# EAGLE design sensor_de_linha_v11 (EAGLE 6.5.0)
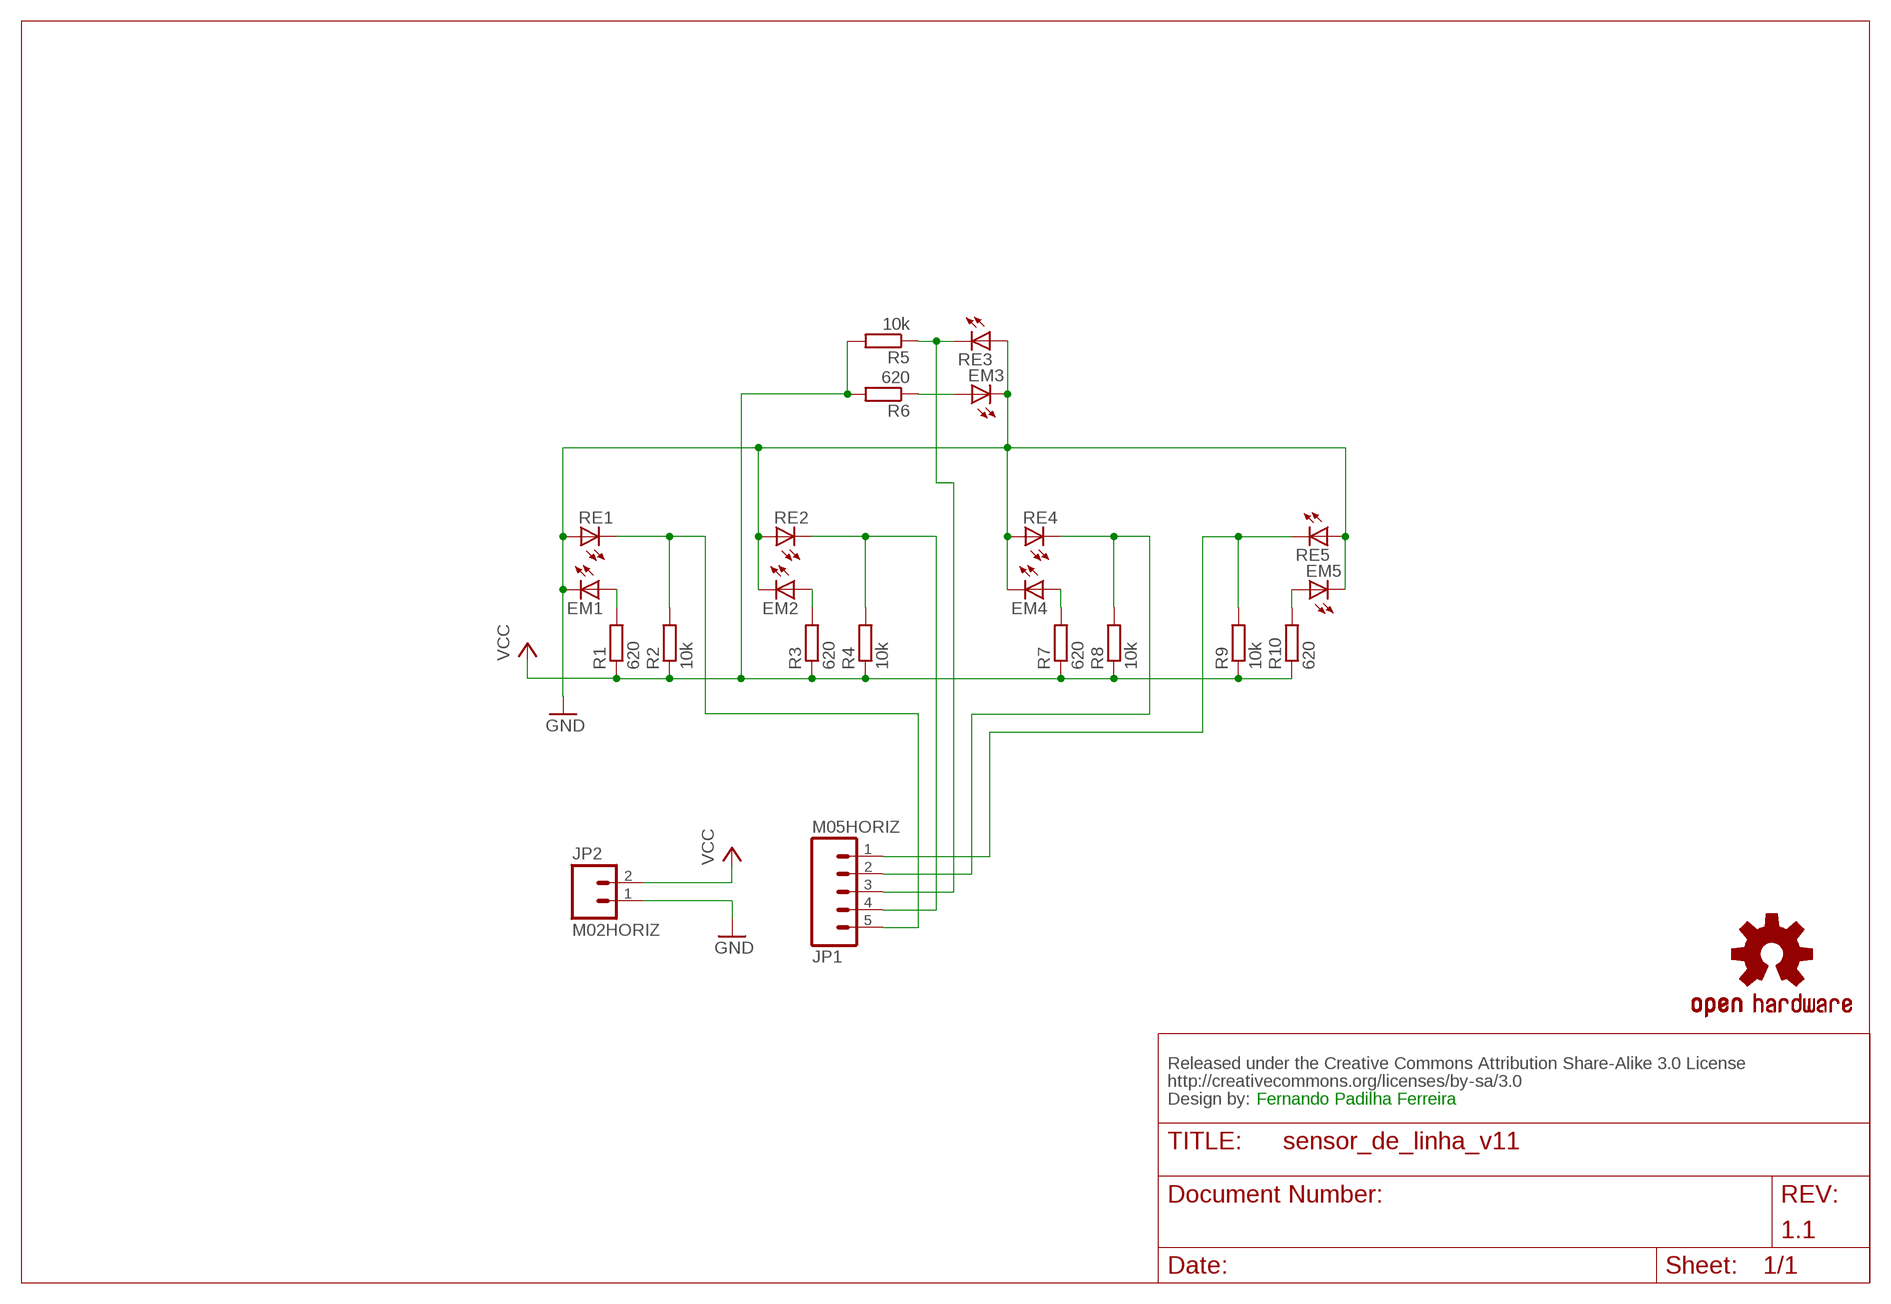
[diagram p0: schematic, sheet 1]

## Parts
CC_TEXT1  CREATIVE_COMMONS  [CREATIVE_COMMONS]
EM1  LED3MM  [LED3MM]
EM2  LED3MM  [LED3MM]
EM3  LED3MM  [LED3MM]
EM4  LED3MM  [LED3MM]
EM5  LED3MM  [LED3MM]
JP1  M05HORIZ  [MOLEX-1X5_HORIZ]
JP2  M02HORIZ  [MOLEX-1X2_HORIZ]
LOGO1  OSHW-LOGOL  [OSHW-LOGO-L]
R1  620  R-EU_0207/7  [0207/7]
R2  10k  R-EU_0207/7  [0207/7]
R3  620  R-EU_0207/7  [0207/7]
R4  10k  R-EU_0207/7  [0207/7]
R5  10k  R-EU_0207/7  [0207/7]
R6  620  R-EU_0207/7  [0207/7]
R7  620  R-EU_0207/7  [0207/7]
R8  10k  R-EU_0207/7  [0207/7]
R9  10k  R-EU_0207/7  [0207/7]
R10  620  R-EU_0207/7  [0207/7]
RE1  LED3MM  [LED3MM]
RE2  LED3MM  [LED3MM]
RE3  LED3MM  [LED3MM]
RE4  LED3MM  [LED3MM]
RE5  LED3MM  [LED3MM]

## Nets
GND: EM1.K(C) EM2.K(C) EM3.K(C) EM4.K(C) EM5.K(C) JP2.1 RE1.A RE2.A RE3.A RE4.A RE5.A
N$1: EM1.A R1.2
N$3: EM2.A R3.2
N$5: EM4.A R7.2
N$7: EM5.A R10.2
N$10: EM3.A R6.1
S1: JP1.5 R2.2 RE1.K(C)
S2: JP1.4 R4.2 RE2.K(C)
S3: JP1.3 R5.1 RE3.K(C)
S4: JP1.2 R8.2 RE4.K(C)
S5: JP1.1 R9.2 RE5.K(C)
VCC: JP2.2 R1.1 R2.1 R3.1 R4.1 R5.2 R6.2 R7.1 R8.1 R9.1 R10.1

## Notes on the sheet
- Fernando Padilha Ferreira
- 1.1

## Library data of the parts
CC_TEXT1 = SparkFun-Aesthetics:CREATIVE_COMMONS: Creative Commons License summary
EM1-EM5 RE1-RE5 = led:LED: LED
JP1 = FernandoLib:M05
JP2 = FernandoLib:M02
LOGO1 = SparkFun-Aesthetics:OSHW-LOGO: Open Source Hardware Logo This logo indicates the piece of hardware it is found on incorporates a OSHW license and/or adheres to the definition of open source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
R1-R10 = resistor:R-EU_: RESISTOR, European symbol

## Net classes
0 default: width 0.406 mm

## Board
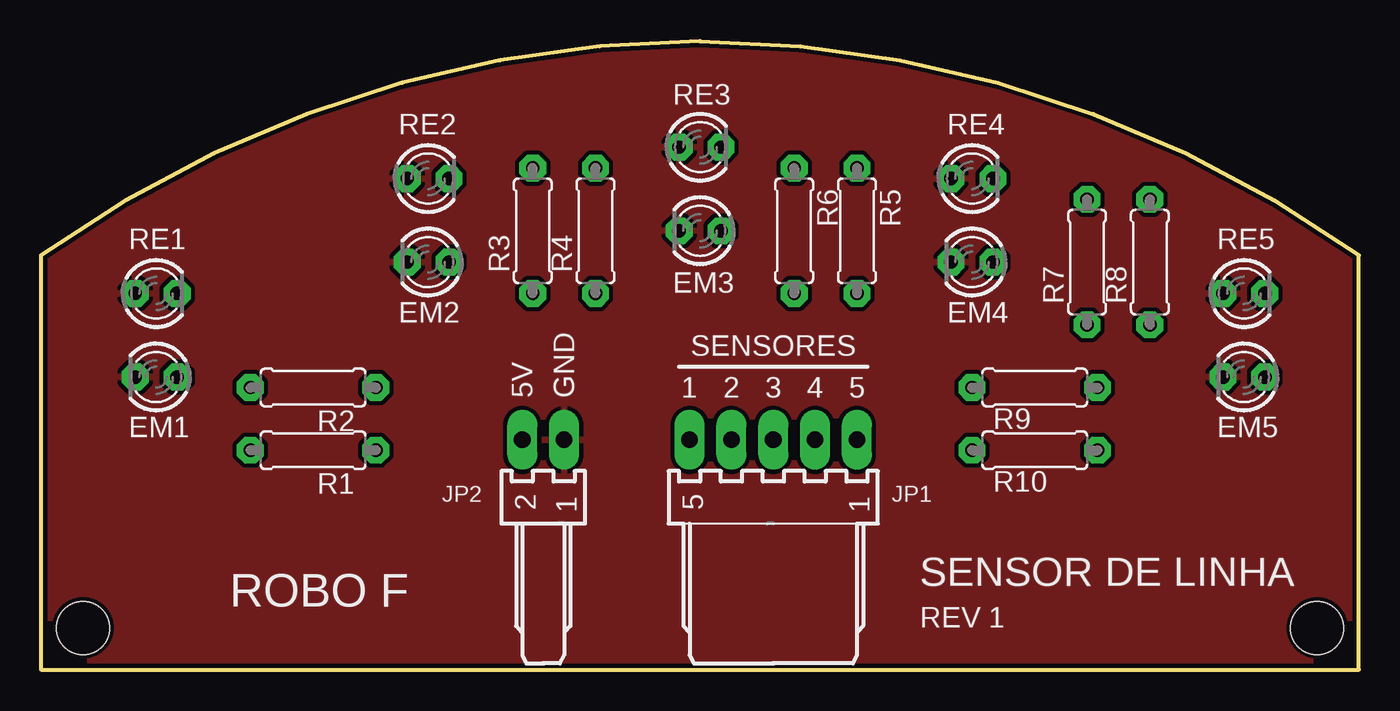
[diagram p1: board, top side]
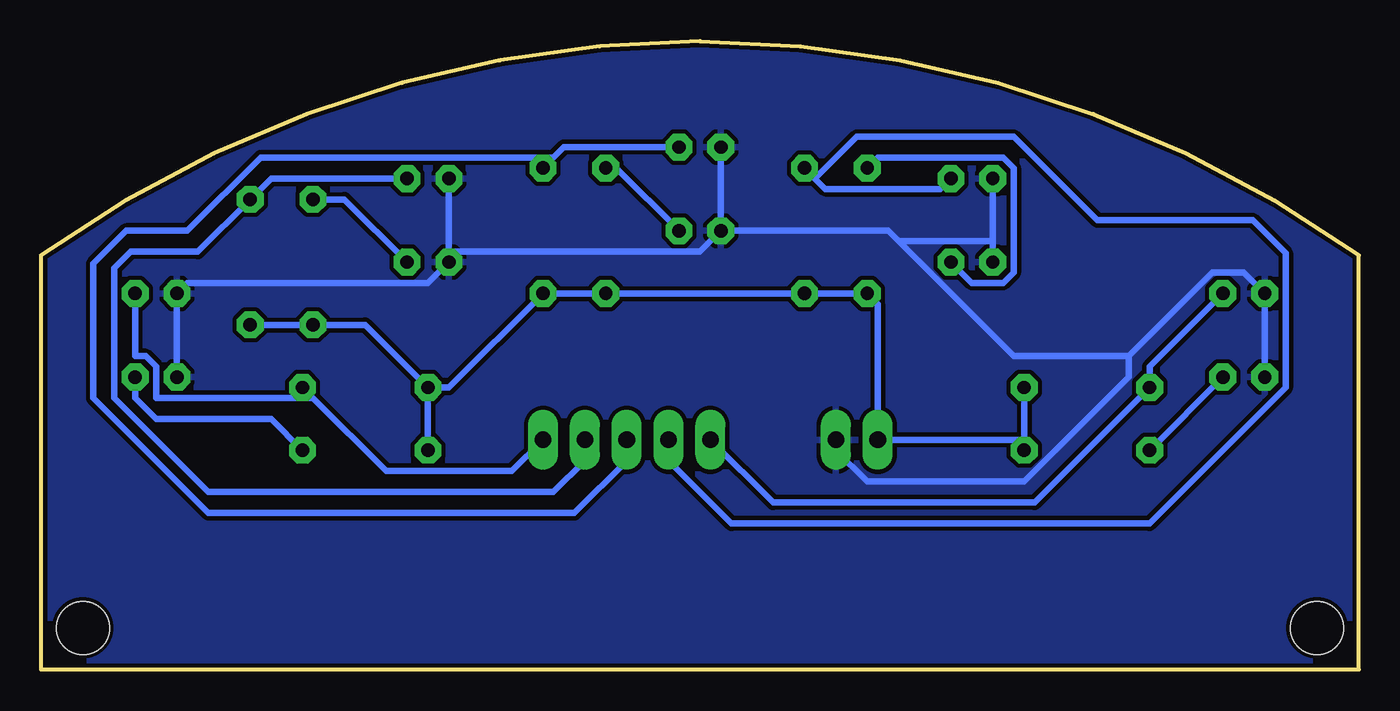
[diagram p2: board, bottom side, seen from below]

Size 80 x 38.19 mm. Coordinates in mm from the lower left corner, seen from the top.
Outline: 0,0 0,25.19 arc-35 40,38.19 arc-35 80,25.19 80,0 0,0
Copper layers (1*16): Top 0.035mm / dielectric 1.5mm / Bottom 0.035mm
Design rules "peteco": minimum track width 12mil, minimum drill 19mil, track to track 10mil, track to pad 10mil, pad to pad 10mil, via to via 10mil, smd to smd 0mil, copper to edge 10mil, drill to drill 8mil, minimum pad ring 16mil, minimum via ring 8mil, stop-mask expansion 4mil, vias tented up to drill 0mil, thermal gap 10mil
Holes 3.2 mm at 2.54,2.54 77.47,2.54

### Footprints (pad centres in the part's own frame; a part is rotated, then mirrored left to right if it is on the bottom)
LED3MM = drill 0.813 octagon: A -1.27,0; K 1.27,0
MOLEX-1X5_HORIZ = drill 1.016 long: 1 0,0; 2 -2.54,0; 3 -5.08,0; 4 -7.62,0; 5 -10.16,0
MOLEX-1X2_HORIZ = drill 1.016 long: 1 0,0; 2 -2.54,0
0207/7 = drill 0.813 octagon: 1 -3.81,0; 2 3.81,0

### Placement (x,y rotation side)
CC_TEXT1  not placed on the board
EM1  6.99,17.78 180 top
EM2  23.5,24.77 180 top
EM3  40.01,26.67 180 top
EM4  56.52,24.77 180 top
EM5  73.03,17.78 180 top
JP1  49.53,13.97 0 top
JP2  31.75,13.97 0 top
LOGO1  not placed on the board
R1  16.51,13.34 180 top
R2  16.51,17.14 180 top
R3  29.84,26.67 90 top
R4  33.66,26.67 90 top
R5  49.53,26.67 270 top
R6  45.72,26.67 270 top
R7  63.5,24.77 90 top
R8  67.31,24.77 90 top
R9  60.33,17.14 0 top
R10  60.33,13.34 0 top
RE1  6.99,22.86 0 top
RE2  23.5,29.84 0 top
RE3  40.01,31.75 0 top
RE4  56.52,29.84 0 top
RE5  73.03,22.86 0 top

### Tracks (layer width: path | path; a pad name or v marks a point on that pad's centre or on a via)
GND
  Bottom 0.406: EM5.K RE5.A 71.12,23.5 56.52,23.5 EM4.K 55.24,25.4 | RE4.A 55.24,25.4 | RE3.A EM3.K | EM1.K RE1.A 6.99,24.13 8.89,24.13 13.97,19.05 | 55.24,25.4 40.01,25.4 EM3.K | JP2.1 31.75,13.34 29.84,11.43 20.32,11.43 13.97,17.78 13.97,19.05 | EM3.K 28.57,26.67 27.94,26.04 | 27.94,26.04 20.95,19.05 13.97,19.05 | RE2.A 22.23,26.04 | 22.23,26.04 EM2.K | 27.94,26.04 22.23,26.04
  pour Top: 0,0 80.01,0 80.01,38.1 0,38.1
  pour Bottom: 0,0 80.01,0 80.01,38.1 0,38.1
N$1
  Bottom 0.406: EM1.A R1.2
N$3
  Bottom 0.406: EM2.A 23.5,23.5 21.59,23.5 20.95,24.13 20.95,30.48 21.59,31.11 29.21,31.11 R3.2
N$5
  Bottom 0.406: EM4.A 61.59,28.57 R7.2
N$7
  Bottom 0.406: R10.2 66.04,15.24 73.03,15.24 74.3,16.51 EM5.A
N$10
  Bottom 0.406: EM3.A 45.09,30.48 R6.1
S1
  Bottom 0.406: RE1.K 12.7,18.41 R2.2 19.68,10.16 35.56,10.16 JP1.5
S2
  Bottom 0.406: RE2.K 25.4,29.21 32.38,29.21 33.02,29.84 | R4.2 33.02,29.84 | JP1.4 41.91,12.7 38.1,8.89 12.7,8.89 4.45,17.14 4.45,25.3 6.45,27.3 15.88,27.3 20.95,32.38 30.48,32.38 33.02,29.84
S3
  Bottom 0.406: 48.9,31.11 48.26,31.75 RE3.K | 48.9,31.11 R5.1 | JP1.3 44.45,12.7 47.62,9.53 69.85,9.53 76.83,16.51 76.83,24.67 74.83,26.67 71.12,26.67 66.67,31.11 48.9,31.11
S4
  Bottom 0.406: RE4.K 66.04,29.84 R8.2 70.48,25.4 74.56,25.4 75.56,24.4 75.56,16.51 69.85,10.79 48.9,10.79 46.99,12.7 JP1.2
S5
  Bottom 0.406: 63.5,16.51 59.05,12.06 51.44,12.06 JP1.1 | 63.5,16.51 R9.2 | RE5.K 74.3,19.05 73.66,19.05 73.03,18.41 73.03,16.51 63.5,16.51
VCC
  Bottom 0.406: R2.1 20.32,13.97 | R9.1 R10.1 | R8.1 R7.1 60.33,20.95 R9.1 | R9.1 55.24,17.14 R5.2 R6.2 R4.1 R3.1 29.21,22.23 JP2.2 20.32,13.97 | 20.32,13.97 R1.1

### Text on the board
tPlace: SENSORES | 5V | GND | 1 | 2 | 3 | 4 | 5 | SENSOR DE LINHA | ROBO F | REV 1
tDocu: Fernando Padilha Ferreira

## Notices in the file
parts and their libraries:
SparkFun-Aesthetics: Licensing: CC v3.0 Share-Alike You are welcome to use this library for commercial purposes.
SparkFun-Aesthetics: Released under the Creative Commons Attribution Share-Alike 3.0 License
SparkFun-Aesthetics: http://creativecommons.org/licenses/by-sa/3.0
